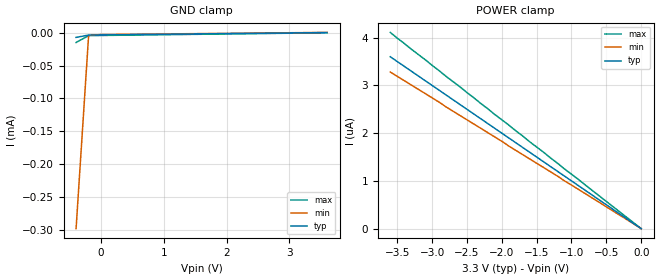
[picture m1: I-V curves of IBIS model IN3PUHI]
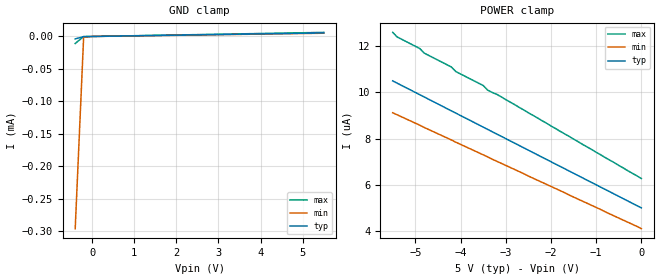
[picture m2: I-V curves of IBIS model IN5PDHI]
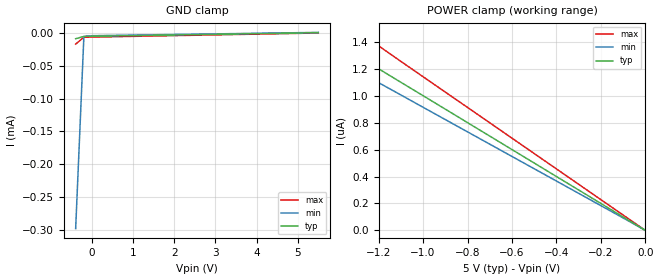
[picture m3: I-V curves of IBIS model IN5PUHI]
|   Texas Instruments Incorporated
|   Data Transmissions Products
|   IBIS Model for ISO723x4x
|   16DW SOIC Package
[IBIS Ver]   3.2
[Comment char]   |_char
[File name]   iso7240cf_53.ibs
[File Rev]   1.0
[Date]   10July08
[Source]   File originated at Texas Instruments Incorporated.
   Data Transmission Products Group.
[Notes]
[Disclaimer]
(C) Copyright Texas Instruments Incorporated 2002
   All rights reserved
  Texas Instruments Incorporated hereby grants the user of this IBIS
model a non-exclusive, nontransferable license to use this IBIS model
under the following terms.  Before using this IBIS model, the user
should read this license.  If the user does not accept these terms,
the IBIS model should be returned to Texas Instruments within 30 days.
  The user is granted this license only to use the IBIS model and
is not granted rights to sell, load, rent, lease or license the IBIS
model in whole or in part, or in modified form to anyone other than
user.  User may modify the IBIS model to suit its specific applications
but rights to derivative works and such modifications shall belong to
Texas Instruments.
  This IBIS model is provided on an "AS IS" basis and Texas Instruments
makes absolutely no warranty with respect to the information contained
herein.  TEXAS INSTRUMENTS DISCLAIMS AND CUSTOMER WAIVES ALL WARRANTIES,
EXPRESS OR IMPLIED, INCLUDING WARRANTIES OF MERCHANTABILITY OR FITNESS
FOR A PARTICULAR PURPOSE. The entire risk as to quality and performance
is with the Customer. ACCORDINGLY, IN NO EVENT SHALL THE COMPANY BE LIABLE
FOR ANY DAMAGES, WHETHER IN CONTRACT OR TORT,INCLUDING ANY LOST PROFITS
OR OTHER INCIDENTAL, CONSEQUENTIAL, EXEMPLARY, OR PUNITIVE DAMAGES ARISING
OUT OF THE USE OR APPLICATION OF THE IBIS model provided in this package.
Further, Texas Instruments reserves the right to discontinue or make changes
without notice to any product herein to improve reliability, function, or
design. Texas Instruments does not convey any license under patent rights
or any other intellectual property rights, including those of third parties.
Contact Texas Instruments at ATTN:DATA TRANSMISSIONS
[Copyright]   Copyright 2002, Texas Instruments, All Rights Reserved
[Component]   ISO7240DW
[Manufacturer]  Texas Instruments Incorporated
[Package]
|   typ   min   max
R_pkg   0.04817   0.03432   0.09530
L_pkg   2.4595nH   1.6904nH   4.7034nH
C_pkg   0.847pF   0.428pF   1.397pF
[Pin]   signal_name   model_name   R_pin   L_pin   C_pin
1   VCC1   POWER   0.03455  3.39778n  0.89677p
2   GND1   GND   0.03432  3.12613n  0.84706p
3   INA   IN5PUHI   0.04265  1.85523n  0.57831p
4   INB   IN5PUHI   0.03948  1.69049n  0.59300p
5   INC   IN5PUHI   0.03943  1.70546n  0.55709p
6   IND   IN5PUHI   0.04257  1.86953n  0.56379p
7   DISABLE   IN5PDHI   0.04783  1.99000n  0.60148p
8   GND1   GND   0.03740  4.70338n  1.39696p
9   GND2   GND   0.03763  4.61305n  1.39587p
10   CTRL   IN3PUHI   0.04703  2.01514n  0.58483p
11   OUTD   OUTPUT3   0.07132  2.45946n  0.43321p
12   OUTC   OUTPUT3   0.06147  2.13194n  0.42769p
13   OUTB   OUTPUT3   0.07288  2.39260n  0.48001p
14   OUTA   OUTPUT3   0.09530  3.03704n  0.47622p
15   GND2   GND   0.04817  4.23145n  0.93567p
16   VCC2   POWER   0.04790  4.51154n  0.99405p
| Models and submodels in the file (4): IN3PUHI (Input), IN5PDHI (Input), IN5PUHI (Input), OUTPUT3 (3-state)
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|   Driver Enable
[Model]   IN3PUHI
Model_type   Input
|Signals   INA,INB,INC,IND,CTRL
Vinh = 2.0
Vinl = 0.8
|   typ   min   max
C_comp   1.3pF   1.1pF   1.5pF
|   typ   min   max
[Temperature Range]   27   -40   125
[Voltage range]   3.3V   3.0V   3.6V
[GND_clamp]
|   Voltage   I(typ)   I(min)   I(max)
-400mV    -7.04uA    -298uA     -14.8uA
-200mV    -3.5uA     -3.91uA    -4.34uA
0V        -3.3uA     -2.74uA    -4.11uA
3.6V      300nA      549nA      14.4pA
[Power_clamp]
| Note that the[POWER_clamp]voltage table is referenced to Vcc
| and is calculated using Vtable=Vcc - Vmeasured.
|   Voltage   I(typ)   I(min)   I(max)
-3.6V     3.6uA      3.28uA     4.11uA
-2.9V     2.9uA      2.65uA     3.31uA
-2.8V     2.8uA      2.55uA     3.19uA
0V        0A         0A         0A
|   Driver Enable
[Model]   IN5PDHI
Model_type   Input
|Signals   DISABLE
Vinh = 2.0
Vinl = 0.8
|   typ   min   max
C_comp   1.3pF   1.1pF   1.5pF
|   typ   min   max
[Temperature Range]   27   -40   85
[Voltage range]   5.0V   4.5V   5.5V
[GND_clamp]
|   Voltage   I(typ)   I(min)   I(max)
-400mV    -3.79uA    -296uA     -10.8uA
-200mV    -202nA     -1.2uA     -230nA
0V        0A         0A         0A
5.5V      5.5uA      5.02uA     6.27uA
[Power_clamp]
| Note that the[POWER_clamp]voltage table is referenced to Vcc
| and is calculated using Vtable=Vcc - Vmeasured.
|   Voltage   I(typ)   I(min)   I(max)
-5.5V     10.5uA     9.12uA     12.6uA
-5.4V     10.4uA     9.03uA     12.4uA
-4.9V     9.9uA      8.58uA     11.9uA
-4.8V     9.8uA      8.48uA     11.7uA
-4.2V     9.2uA      7.94uA     11.1uA
-4.1V     9.1uA      7.84uA     10.9uA
-3.5V     8.5uA      7.3uA      10.3uA
-3.4V     8.4uA      7.21uA     10.1uA
-3.1V     8.1uA      6.93uA     9.81uA
0V        5uA        4.1uA      6.27uA
|   Driver Input / Receiver Enable Model
[Model]   IN5PUHI
Model_type   Input
|Signals   INA,INB,INC,IND,EN
Vinh = 2.0
Vinl = 0.8
|   typ   min   max
C_comp   1.3pF   1.1pF   1.5pF
|   typ   min   max
[Temperature Range]   27   -40   125
[Voltage range]   5.0V   4.5V   5.5V
[GND_clamp]
|   Voltage   I(typ)   I(min)   I(max)
-400mV    -8.71uA    -298uA     -16.9uA
-200mV    -5.2uA     -5.27uA    -6.5uA
0V        -5uA       -4.1uA     -6.27uA
5.5V      500nA      913nA      27.5pA
[Power_clamp]
| Note that the[POWER_clamp]voltage table is referenced to Vcc
| and is calculated using Vtable=Vcc - Vmeasured.
|   Voltage   I(typ)   I(min)   I(max)
-5.5V     5.498uA    5.021uA    6.28uA
-1.7V     1.699uA    1.552uA    1.939uA
-1.6V     1.599uA    1.461uA    1.825uA
-1.5V     1.499uA    1.369uA    1.711uA
-1.4V     1.399uA    1.278uA    1.597uA
-1.3V     1.299uA    1.187uA    1.483uA
0V        0A         0A         0A
